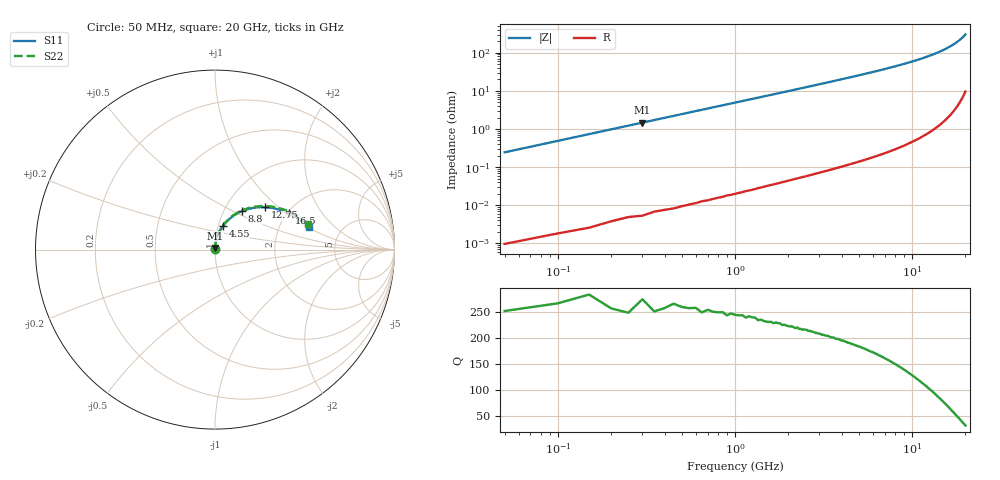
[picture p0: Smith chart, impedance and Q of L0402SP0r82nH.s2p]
!	AVX Thin Film Operation
!	Date:		5 January 2004
!	Description: 	Accu-L®  L0402 Series Thin Film RF Inductors
!	Part Number:	L0402R82AHLTR
!	50 MHz-20GHz Serial Measurements
#	mhz	S	db	R	50
!	S11	S11	S21	S21	S12	S12	S22	S22
!	dB	Phase	dB	Phase	dB	Phase	dB	Phase
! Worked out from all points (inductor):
!   400 points, 50 MHz to 20 GHz, reference 50 ohm
!   read as 1/Y11, port 2 shorted: L = 778 pH near 150 MHz
!   highest Q = 260 at 300 MHz (marker M1), where L = 778 pH
!   S11 on the Smith chart (normalised r, x): 50 MHz: 1.00, +0.00; 4.55 GHz: 1.05, +0.28; 8.8 GHz: 1.21, +0.55; 12.75 GHz: 1.51, +0.82; 16.5 GHz: 2.05, +1.05; 20 GHz: 2.92, +1.02
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50  -56.41 89.5  -0.00 -0.2  -0.00 -0.2  -56.41 89.5
100  -50.39 89.3  -0.00 -0.4  -0.00 -0.4  -50.39 89.3
150  -46.87 89.1  -0.00 -0.6  -0.00 -0.6  -46.87 89.1
200  -44.37 88.9  -0.00 -0.8  -0.00 -0.8  -44.37 88.9
300  -40.85 88.5  -0.00 -1.2  -0.00 -1.2  -40.85 88.5
450  -37.32 87.9  -0.00 -1.7  -0.00 -1.7  -37.32 87.9
550  -35.58 87.5  -0.00 -2.1  -0.00 -2.1  -35.58 87.5
700  -33.49 86.9  -0.00 -2.7  -0.00 -2.7  -33.49 87.0
950  -30.83 85.9  -0.01 -3.7  -0.01 -3.7  -30.83 86.0
1300  -28.11 84.5  -0.01 -5.0  -0.01 -5.0  -28.11 84.7
1700  -25.78 82.9  -0.01 -6.6  -0.01 -6.6  -25.78 83.1
2200  -23.55 80.9  -0.02 -8.5  -0.02 -8.5  -23.55 81.2
3400  -19.78 76.2  -0.05 -13.1  -0.05 -13.1  -19.78 76.6
4550  -17.27 71.7  -0.09 -17.6  -0.09 -17.6  -17.27 72.2
6700  -13.98 63.3  -0.19 -25.8  -0.19 -25.8  -13.98 64.0
8800  -11.70 55.1  -0.33 -33.8  -0.33 -33.8  -11.70 56.1
10050  -10.61 50.3  -0.42 -38.6  -0.42 -38.6  -10.61 51.4
12750  -8.71 40.0  -0.67 -48.6  -0.67 -48.6  -8.71 41.4
13350  -8.35 37.8  -0.73 -50.8  -0.73 -50.8  -8.35 39.2
16500  -6.75 26.1  -1.09 -62.3  -1.09 -62.3  -6.75 27.8
16700  -6.67 25.3  -1.11 -63.0  -1.11 -63.0  -6.67 27.1
20000  -5.40 13.4  -1.56 -74.7  -1.56 -74.7  -5.40 15.5
